(* 	
	Program Name: 	ACS_SAMPLE_INDEXED_MOVES
	Purpose:		Example of a program that executes a series of moves defined in the index table of the drive (done in TMI)
	When Executed:	Executes a specified index, waits for that move to complete, then executes the next move in the index table
*)
PROGRAM ACS_SAMPLE_INDEXED_MOVES
VAR_IN_OUT 
	Axis:ACS_DRIVE_TYPE;
END_VAR

VAR
	_readyToRumble	:BOOL;
	_currentIndex	:USINT	:= 1;
END_VAR

(* 
	This program contains both the input and output scan and is intented to be a stand alone application
	Remember : The input scan should be one of the first things done in the program.  Then the processing.  
	Then the Output Scan.
	|->Input Scan
	|
	|->Processing (User Code)
	|
	|->Output Scan
*)

//Input Scan Routine
ACS_DRIVE_INPUT_SCAN(Axis:=Axis);

//Processing (User Code)

//Step 1. Initialize the drive
ACS_INITIALIZATION_NOBRAKE(Axis:=Axis);

//Step 2. Determine if we are Ready To Rumble (motion is possible)
_readyToRumble := (Axis.InputStatusDriveEnabled AND Axis.InputStatusDriveHomed AND NOT Axis.InputFaultActive);	

//Step 4. Run program based on extend or retracted state
IF _readyToRumble THEN
	
	//In Motion
	IF Axis.InputStatusDriveInMotion THEN
		IF Axis.OutputCommand = ACS_COMMANDS.START_MOTION THEN
			_currentIndex := _currentIndex + 1; //Only should do this once, we will reset command on the way through
			IF _currentIndex > 16 THEN
				_currentIndex := 1;
			END_IF
		END_IF
		ACS_CMD_CLEAR_START_MOTION(Axis := Axis);
	ELSE	// Not In Motion
		ACS_MOVE_INDEXED(Axis := Axis, IndexPosition := _currentIndex);
		ACS_CMD_START_MOTION(Axis := Axis);	
	END_IF
	
END_IF

//End processing (User Code)

//Output Scan Routine
ACS_DRIVE_OUTPUT_SCAN(Axis:=Axis);

END_PROGRAM
